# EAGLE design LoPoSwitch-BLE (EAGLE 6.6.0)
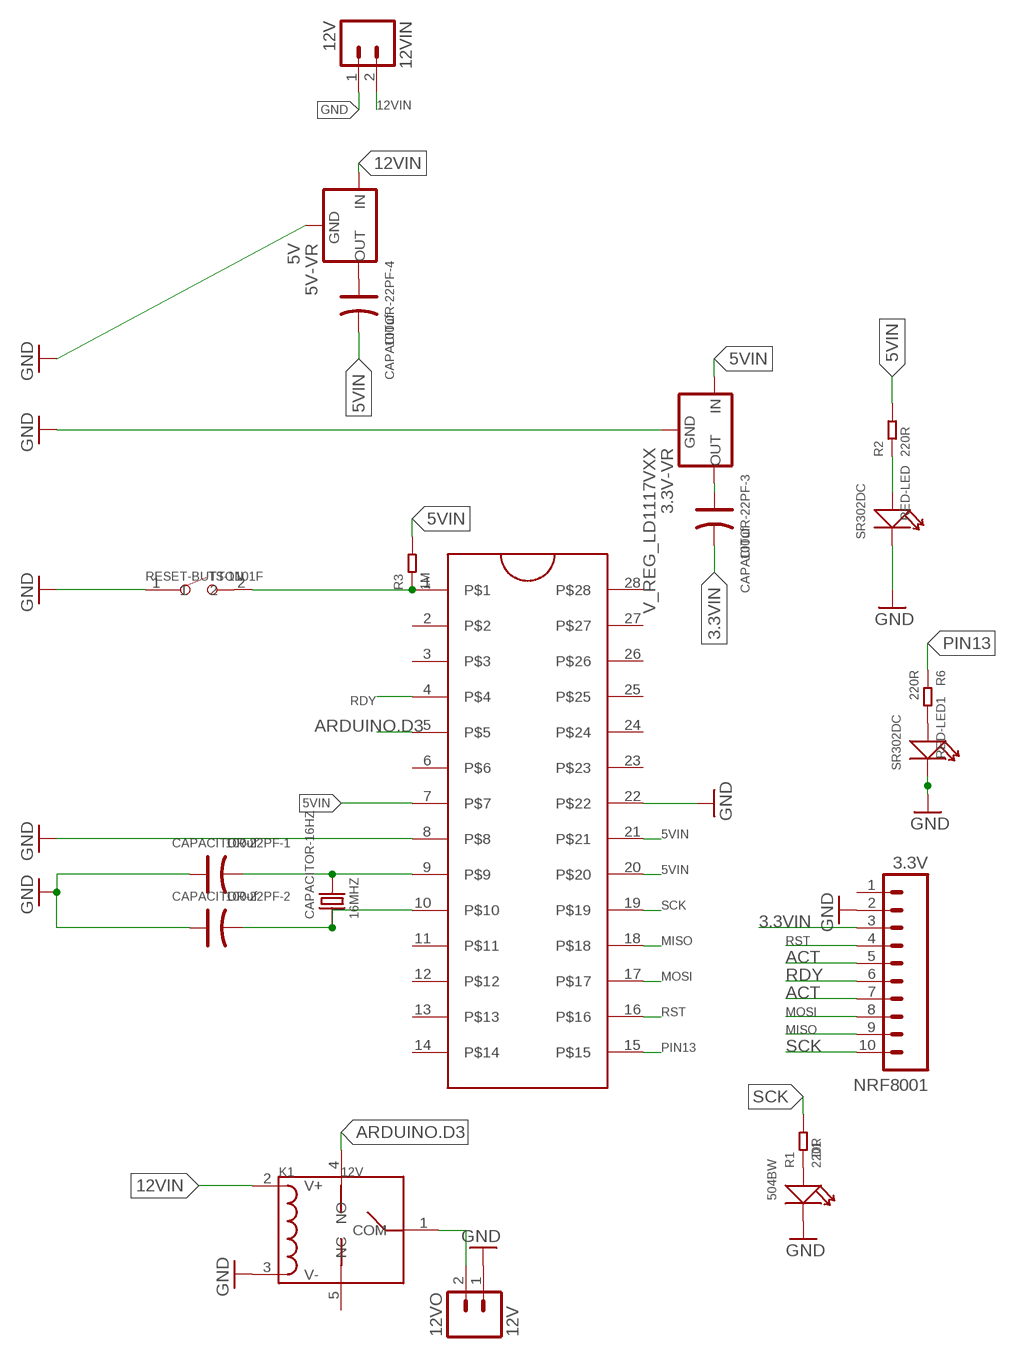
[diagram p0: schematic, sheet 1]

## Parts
3.3V-VR  V_REG_LD1117VXX  [78XXL]
5V-VR  5V  V_REG_78XX-TO-220  [TO-220-ALT]
12VIN  12V  M02JST-PTH-2  [JST-2-PTH]
12VO  12V  M02JST-PTH-2  [JST-2-PTH]
ATMEGA328  ZIFSOCKET-28-3ZIFFSOCKET-28-3  [DIL28-3-ZIF_SOCKET]
CAPACITOR-16HZ  16MHZ  DIP-CRYSTAL-16MHZ-18PF-30PPM-50R(HC49US)  [HC49US]
CAPACITOR-22PF-1  100uf  DIP-ALUMINUM-47UF-16V(D5-H7MM)  [PC-D5.3MM]
CAPACITOR-22PF-2  100uf  DIP-ALUMINUM-47UF-16V(D5-H7MM)  [PC-D5.3MM]
CAPACITOR-22PF-3  100uf  DIP-ALUMINUM-47UF-16V(D5-H7MM)  [PC-D5.3MM]
CAPACITOR-22PF-4  100uf  DIP-ALUMINUM-47UF-16V(D5-H7MM)  [PC-D5.3MM]
D1  504BW  DIP-LED-BLUE-BLUE(2P-D5MM)  [LED2-2.54-D5.0MM]
K1  12V  RELAY-HLS8L-DC5V-S-CHLS8L-DC5V-S-C  [REY5-19.0X15.0X15.0MM]
NRF8001  3.3V  M10SILK_FEMALE_PTH  [1X10]
R1  220R  DIP-RES-220R-5%-1/4W(PR-D2.3XL6.5MM)  [PR-D2.3XL6.5MM]
R2  220R  DIP-RES-220R-5%-1/4W(PR-D2.3XL6.5MM)  [PR-D2.3XL6.5MM]
R3  1M  DIP-RES-1M-5%-1/4W(PR-D2.3XL6.5MM)  [PR-D2.3XL6.5MM]
R6  220R  DIP-RES-220R-5%-1/4W(PR-D2.3XL6.5MM)  [PR-D2.3XL6.5MM]
RED-LED  SR302DC  DIP-LED-RED-RED(2P-D3MM)  [LED2-2.54-D3.0MM]
RED-LED1  SR302DC  DIP-LED-RED-RED(2P-D3MM)  [LED2-2.54-D3.0MM]
RESET-BUTTON  TS-1101F  DIP-BUTTON(2P-6.0X3.0X4.3MM)-TS-1101F  [SW2-5.0-6.0X3.0X4.3MM]

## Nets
3.3VIN: CAPACITOR-22PF-3.- NRF8001.3
5VIN: 3.3V-VR.OUT(IN) ATMEGA328.7 ATMEGA328.20 ATMEGA328.21 CAPACITOR-22PF-4.- R2.2 R3.2
12VIN: 5V-VR.IN 12VIN.2 K1.2(V+)
ACT: NRF8001.5 NRF8001.7
ARDUINO.D3: ATMEGA328.5 K1.4(NO)
GND: 3.3V-VR.IN(GND) 5V-VR.GND 12VIN.1 12VO.1 ATMEGA328.8 ATMEGA328.22 CAPACITOR-22PF-1.+ CAPACITOR-22PF-2.+ D1.- K1.3(V-) NRF8001.2 RED-LED1.K(-) RED-LED.K(-) RESET-BUTTON.1
MISO: ATMEGA328.18 NRF8001.9
MOSI: ATMEGA328.17 NRF8001.8
N$1: 12VO.2 K1.1(COM)
N$2: R6.2 RED-LED1.A(+)
N$3: ATMEGA328.1 R3.1 RESET-BUTTON.2
N$4: 3.3V-VR.GND(OUT) CAPACITOR-22PF-3.+
N$5: 5V-VR.OUT CAPACITOR-22PF-4.+
N$7: D1.+ R1.1
N$8: R2.1 RED-LED.A(+)
N$10: ATMEGA328.9 CAPACITOR-16HZ.2 CAPACITOR-22PF-1.-
N$11: ATMEGA328.10 CAPACITOR-16HZ.1 CAPACITOR-22PF-2.-
PIN13: ATMEGA328.15 R6.1
RDY: ATMEGA328.4 NRF8001.6
RST: ATMEGA328.16 NRF8001.4
SCK: ATMEGA328.19 NRF8001.10 R1.2
Unconnected: ATMEGA328.2 ATMEGA328.3 ATMEGA328.6 ATMEGA328.11 ATMEGA328.12 ATMEGA328.13 ATMEGA328.14 ATMEGA328.23 ATMEGA328.24 ATMEGA328.25 ATMEGA328.26 ATMEGA328.27 ATMEGA328.28 K1.5(NC) NRF8001.1

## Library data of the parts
3.3V-VR = SparkFun-PowerIC:V_REG_LD1117VXX: LD1117VXX voltage regulator. We carry the 3.3V version (COM-00526) in TO-220 package.
5V-VR = SparkFun-PowerIC:V_REG_78XX: Voltage Regulator Standard 78xx regulator. IGO (Input Ground Output). Spark Fun Electronics SKU : COM-00107; PROD_ID: VREG-08450; SF_ID: COM-00107
12VIN 12VO = SparkFun-Connectors:M02: Standard 2-pin 0.1" header. Use with; PROD_ID: CONN-09863; SKU: PRT-09914
ATMEGA328 = SparkFun-Connectors:ZIFSOCKET-28-3: Lever-action ZIF socket for 28-pin ICs
CAPACITOR-16HZ = Seeed-Crystal Oscillator:DIP-CRYSTAL-16MHZ-18PF-30PPM-50R(HC49US): 306010037; MPN: 49S/18PF
CAPACITOR-22PF-1-CAPACITOR-22PF-4 = Seeed-Capacitor:DIP-ALUMINUM-47UF-16V(D5-H7MM): 302030033; MPN: KS 100uF/16V
D1 = Seeed-LED:DIP-LED-BLUE-BLUE(2P-D5MM): 304090062; MPN: 504BW
K1 = Seeed-Relay:RELAY-HLS8L-DC5V-S-C: 315030000
NRF8001 = SparkFun-Connectors:M10: Header 10 Standard 10-pin 0.1" header. Use with straight break away headers (SKU : PRT-00116), right angle break away headers (PRT-00553), swiss pins (PRT-00743), machine pins (PRT-00117), and female headers (PRT-00115).; PROD_ID: CONN-11563
R1 R2 R6 = Seeed-Resistor:DIP-RES-220R-5%-1/4W(PR-D2.3XL6.5MM): 301020011; MPN: FHCFR-1/4W-221J
R3 = Seeed-Resistor:DIP-RES-1M-5%-1/4W(PR-D2.3XL6.5MM): 301020005; MPN: FHCFR-1/4W-105J
RED-LED RED-LED1 = Seeed-LED:DIP-LED-RED-RED(2P-D3MM): 304090041; MPN: SR302DC
RESET-BUTTON = Seeed-Switch:DIP-BUTTON(2P-6.0X3.0X4.3MM): 311020025; MPN: TS-1101F

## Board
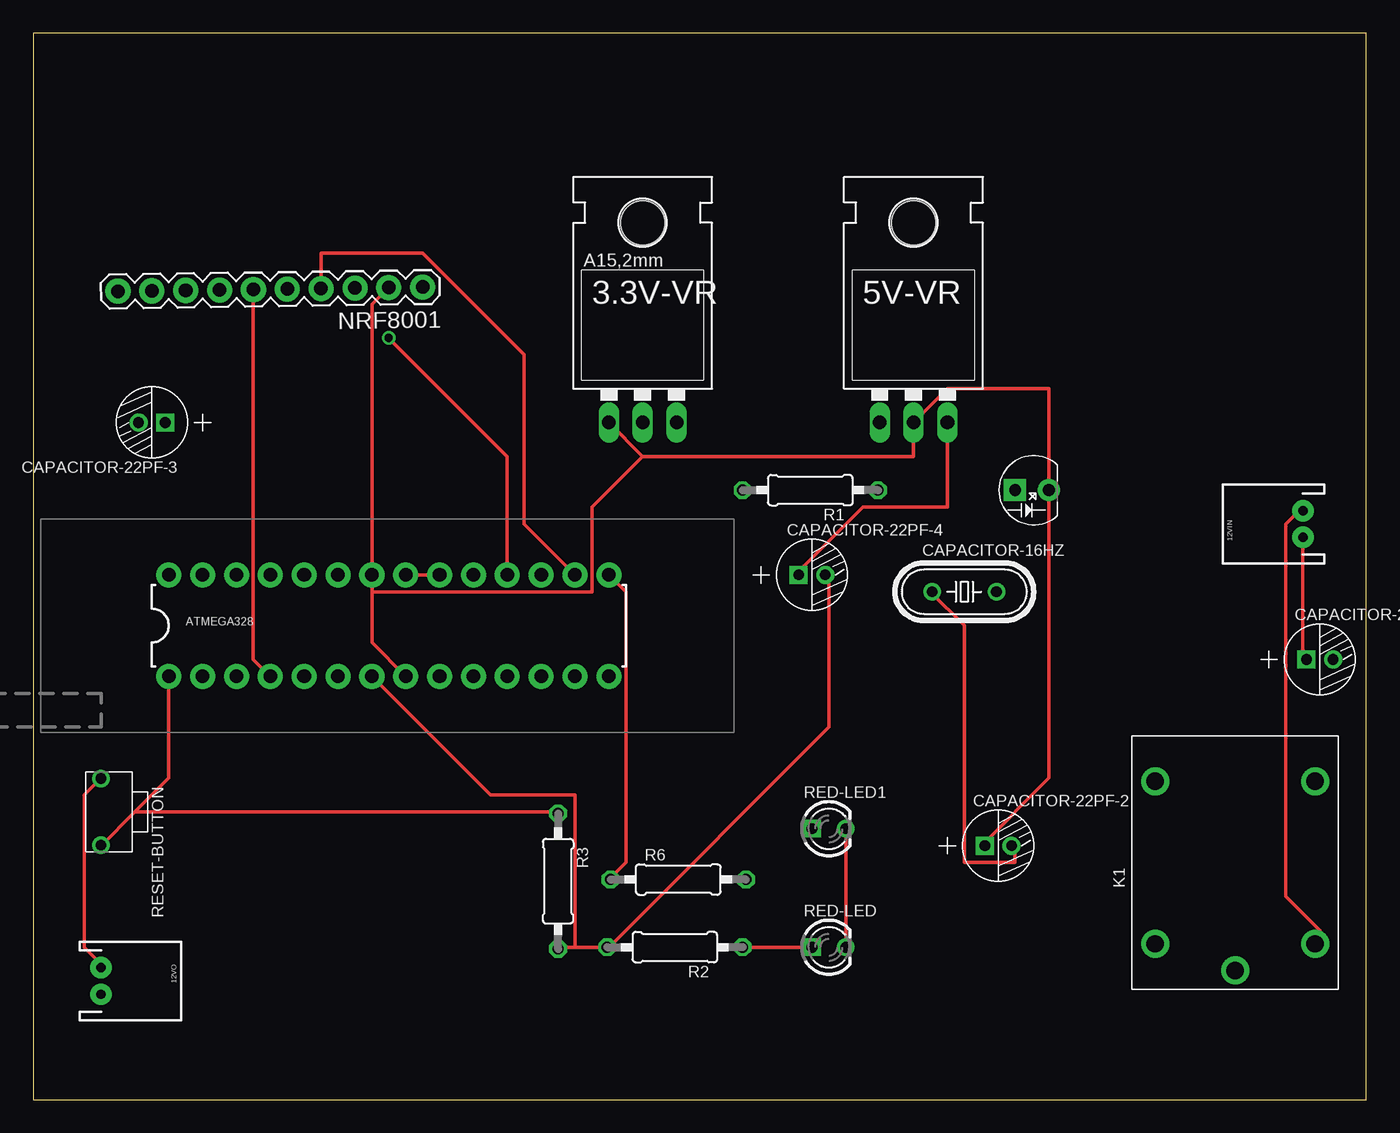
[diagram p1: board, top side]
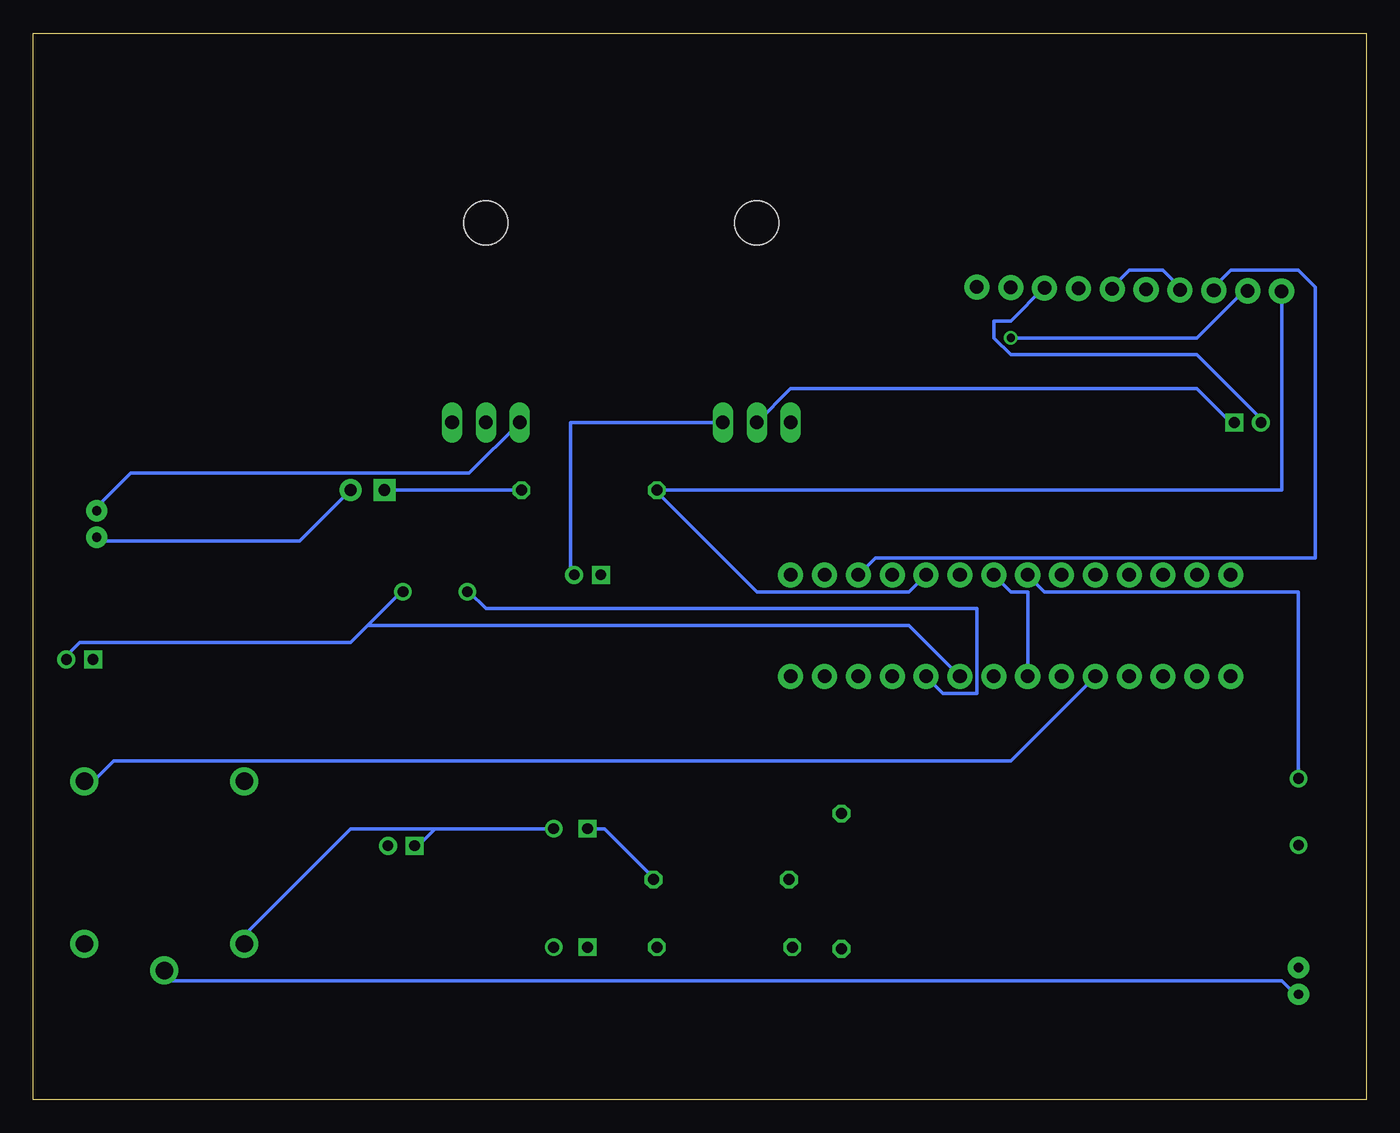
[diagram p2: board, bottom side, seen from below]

Size 100 x 80 mm. Coordinates in mm from the lower left corner, seen from the top.
Outline: 0,0 100,0 100,80 0,80 0,0
Copper layers (1*16): Top 0.035mm / dielectric 1.5mm / Bottom 0.035mm
Design rules "default": minimum track width 10mil, minimum drill 24mil, track to track 8mil, track to pad 8mil, pad to pad 8mil, via to via 8mil, smd to smd 8mil, copper to edge 40mil, drill to drill 8mil, minimum pad ring 10mil, minimum via ring 8mil, stop-mask expansion 4mil, vias tented up to drill 0mil, thermal gap 10mil

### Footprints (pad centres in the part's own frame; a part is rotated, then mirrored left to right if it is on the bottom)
78XXL = drill 1.016 long: GND 0,-3.81; IN -2.54,-3.81; OUT 2.54,-3.81 | hole 3.302: 0,11.176
TO-220-ALT = drill 1.016 long: GND 0,-3.81; IN -2.54,-3.81; OUT 2.54,-3.81 | hole 3.302: 0,11.176
JST-2-PTH = drill 0.7 pad 1.6: 1 -1,0; 2 1,0
DIL28-3-ZIF_SOCKET = drill 1.016 pad 1.88: 1 -16.51,-3.81; 2 -13.97,-3.81; 3 -11.43,-3.81; 4 -8.89,-3.81; 5 -6.35,-3.81; 6 -3.81,-3.81; 7 -1.27,-3.81; 8 1.27,-3.81; 9 3.81,-3.81; 10 6.35,-3.81; 11 8.89,-3.81; 12 11.43,-3.81; 13 13.97,-3.81; 14 16.51,-3.81; 15 16.51,3.81; 16 13.97,3.81; 17 11.43,3.81; 18 8.89,3.81; 19 6.35,3.81; 20 3.81,3.81; 21 1.27,3.81; 22 -1.27,3.81; 23 -3.81,3.81; 24 -6.35,3.81; 25 -8.89,3.81; 26 -11.43,3.81; 27 -13.97,3.81; 28 -16.51,3.81
HC49US = drill 0.813: 1 -2.413,0; 2 2.413,0
PC-D5.3MM = drill 0.8 pad 1.35 square: + -1,0 | drill 0.8 pad 1.35: - 1,0
LED2-2.54-D5.0MM = drill 0.889 pad 1.651 square: + -1.27,0 | drill 0.889 pad 1.651: - 1.27,0
REY5-19.0X15.0X15.0MM = drill 1.3 pad 2.1: 1 -8.1,0; 2 -6.1,-6; 3 -6.1,6; 4 6.1,-6; 5 6.1,6
1X10 = drill 1.016 pad 1.88: 1 0,0; 2 2.54,0; 3 5.08,0; 4 7.62,0; 5 10.16,0; 6 12.7,0; 7 15.24,0; 8 17.78,0; 9 20.32,0; 10 22.86,0
PR-D2.3XL6.5MM = drill 0.813 octagon: 1 -4.953,0; 2 5.207,0
LED2-2.54-D3.0MM = drill 0.813 square: A -1.27,0 | drill 0.813: K 1.27,0
SW2-5.0-6.0X3.0X4.3MM = drill 0.8 pad 1.27: 1 -2.5,0; 2 2.5,0

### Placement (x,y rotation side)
3.3V-VR  45.72,54.61 0 top
5V-VR  66.04,54.61 0 top
12VIN  95.25,43.18 90 top
12VO  5.08,8.89 270 top
ATMEGA328  26.67,35.56 0 top
CAPACITOR-16HZ  69.85,38.1 0 top
CAPACITOR-22PF-1  96.52,33.02 0 top
CAPACITOR-22PF-2  72.39,19.05 0 top
CAPACITOR-22PF-3  8.89,50.8 180 top
CAPACITOR-22PF-4  58.42,39.37 0 top
D1  74.93,45.72 0 top
K1  90.17,17.78 90 top
NRF8001  29.21,60.96 180.8 top
R1  58.42,45.72 180 top
R2  48.26,11.43 180 top
R3  39.37,16.51 270 top
R6  48.26,16.51 0 top
RED-LED  59.69,11.43 0 top
RED-LED1  59.69,20.32 0 top
RESET-BUTTON  5.08,21.59 270 top

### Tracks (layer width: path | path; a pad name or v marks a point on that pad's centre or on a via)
3.3VIN
  Bottom 0.254: CAPACITOR-22PF-3.- 7.62,50.8 12.7,55.88 26.67,55.88 27.94,57.15 27.94,58.42 26.67,58.42 24.13,60.96 NRF8001.3
5VIN
  Top 0.254: ATMEGA328.21 ATMEGA328.20 | 40.64,11.43 R2.2 43.18,11.43 59.69,27.94 59.69,39.37 CAPACITOR-22PF-4.- | 40.64,11.43 39.37,11.43 R3.2 | ATMEGA328.7 34.29,22.86 40.64,22.86 40.64,11.43
  Bottom 0.254: ATMEGA328.7 25.4,38.1 26.67,38.1 ATMEGA328.21 | 3.3V-VR.OUT 59.69,50.8 59.69,39.37 CAPACITOR-22PF-4.-
12VIN
  Top 0.254: K1.2 96.52,12.7 93.98,15.24 93.98,43.18 95.25,44.45 12VIN.2
  Bottom 0.254: 5V-VR.IN 67.31,46.99 92.71,46.99 95.25,44.45 12VIN.2
ACT
  Bottom 0.254: NRF8001.7 13.97,60.96 15.24,62.23 17.78,62.23 19.05,60.96 NRF8001.5
ARDUINO.D3
  Bottom 0.254: ATMEGA328.5 26.67,25.4 93.98,25.4 95.25,24.13 K1.4
GND
  Top 0.254: RESET-BUTTON.1 5.08,24.13 3.81,22.86 3.81,11.43 5.08,10.16 12VO.1 | ATMEGA328.8 25.4,34.29 25.4,38.1 | 25.4,38.1 ATMEGA328.22 25.4,59.69 26.67,60.96 NRF8001.2 | RED-LED1.K RED-LED.K | 45.72,48.26 3.3V-VR.IN | 45.72,48.26 66.04,48.26 5V-VR.GND 68.58,53.34 76.2,53.34 D1.- | 12VIN.1 95.25,33.02 CAPACITOR-22PF-1.+ | D1.- 76.2,24.13 71.12,19.05 CAPACITOR-22PF-2.+ | D1.- | 25.4,38.1 41.91,38.1 41.91,44.45 45.72,48.26
  Bottom 0.254: RESET-BUTTON.1 5.08,38.1 24.13,38.1 ATMEGA328.22 | 69.85,20.32 71.12,19.05 CAPACITOR-22PF-2.+ | RED-LED1.K 69.85,20.32 | 69.85,20.32 76.2,20.32 83.82,12.7 K1.3 | D1.- 80.01,41.91 95.25,41.91 12VIN.1 | D1.-
MISO  (via drill 0.61)
  Top 0.254: v26.67,57.15 35.56,48.26 ATMEGA328.18
  Bottom 0.254: v26.67,57.15 12.7,57.15 8.89,60.96 NRF8001.9
MOSI
  Bottom 0.254: ATMEGA328.17 36.83,40.64 3.81,40.64 3.81,60.96 5.08,62.23 10.16,62.23 11.43,60.96 NRF8001.8
N$1
  Bottom 0.254: 12VO.2 5.08,7.62 6.35,8.89 90.17,8.89 K1.1
N$2
  Bottom 0.254: RED-LED1.A 57.15,20.32 53.34,16.51 R6.2
N$3
  Top 0.254: 7.62,21.59 10.16,24.13 ATMEGA328.1 | 7.62,21.59 5.08,19.05 RESET-BUTTON.2 | 7.62,21.59 39.37,21.59 R3.1
N$4
  Bottom 0.254: 3.3V-VR.GND 43.18,53.34 12.7,53.34 10.16,50.8 CAPACITOR-22PF-3.+
N$5
  Top 0.254: 5V-VR.OUT 68.58,44.45 62.23,44.45 57.15,39.37 CAPACITOR-22PF-4.+
N$7
  Bottom 0.254: D1.+ R1.1
N$8
  Top 0.254: RED-LED.A R2.1
N$10
  Bottom 0.254: 74.93,35.56 76.2,34.29 96.52,34.29 97.79,33.02 CAPACITOR-22PF-1.- | 74.93,35.56 72.39,38.1 CAPACITOR-16HZ.2 | ATMEGA328.9 34.29,35.56 74.93,35.56
N$11
  Top 0.254: CAPACITOR-16HZ.1 67.31,38.1 69.85,35.56 69.85,17.78 73.66,17.78 73.66,19.05 CAPACITOR-22PF-2.-
  Bottom 0.254: ATMEGA328.10 31.75,30.48 29.21,30.48 29.21,36.83 66.04,36.83 67.31,38.1 CAPACITOR-16HZ.1
PIN13
  Top 0.254: ATMEGA328.15 44.45,38.1 44.45,17.78 43.18,16.51 R6.1
RDY
  Top 0.254: ATMEGA328.4 16.51,33.02 16.51,60.96 NRF8001.6
RST
  Top 0.254: ATMEGA328.16 36.83,43.18 36.83,55.88 29.21,63.5 21.59,63.5 21.59,60.96 NRF8001.4
SCK
  Bottom 0.254: ATMEGA328.19 34.29,38.1 45.72,38.1 53.34,45.72 R1.2 6.35,45.72 6.35,60.96 NRF8001.10

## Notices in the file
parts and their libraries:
SparkFun-Connectors: Licensing: Creative Commons ShareAlike 4.0 International - https://creativecommons.org/licenses/by-sa/4.0
